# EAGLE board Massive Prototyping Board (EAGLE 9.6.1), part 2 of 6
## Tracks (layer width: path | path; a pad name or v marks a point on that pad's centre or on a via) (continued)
N$298  (via drill 0.94) (continued)
  Bottom 2.032: v80.01,48.26 v82.55,48.26 v85.09,48.26 v87.63,48.26 v90.17,48.26
N$299  (via drill 0.94)
  Bottom 2.032: v80.01,50.8 v82.55,50.8 v85.09,50.8 v87.63,50.8 v90.17,50.8
N$300  (via drill 0.94)
  Bottom 2.032: v80.01,53.34 v82.55,53.34 v85.09,53.34 v87.63,53.34 v90.17,53.34
N$301  (via drill 0.94)
  Bottom 2.032: v80.01,55.88 v82.55,55.88 v85.09,55.88 v87.63,55.88 v90.17,55.88
N$302  (via drill 0.94)
  Bottom 2.032: v80.01,58.42 v82.55,58.42 v85.09,58.42 v87.63,58.42 v90.17,58.42
N$303  (via drill 0.94)
  Bottom 2.032: v80.01,60.96 v82.55,60.96 v85.09,60.96 v87.63,60.96 v90.17,60.96
N$304  (via drill 0.94)
  Bottom 2.032: v80.01,63.5 v82.55,63.5 v85.09,63.5 v87.63,63.5 v90.17,63.5
N$305  (via drill 0.94)
  Bottom 2.032: v80.01,66.04 v82.55,66.04 v85.09,66.04 v87.63,66.04 v90.17,66.04
N$306  (via drill 0.94)
  Bottom 2.032: v80.01,68.58 v82.55,68.58 v85.09,68.58 v87.63,68.58 v90.17,68.58
N$307  (via drill 0.94)
  Bottom 2.032: v80.01,71.12 v82.55,71.12 v85.09,71.12 v87.63,71.12 v90.17,71.12
N$308  (via drill 0.94)
  Bottom 2.032: v80.01,73.66 v82.55,73.66 v85.09,73.66 v87.63,73.66 v90.17,73.66
N$309  (via drill 0.94)
  Bottom 2.032: v80.01,76.2 v82.55,76.2 v85.09,76.2 v87.63,76.2 v90.17,76.2
N$310  (via drill 0.94)
  Bottom 2.032: v80.01,78.74 v82.55,78.74 v85.09,78.74 v87.63,78.74 v90.17,78.74
N$311  (via drill 0.94)
  Bottom 2.032: v80.01,81.28 v82.55,81.28 v85.09,81.28 v87.63,81.28 v90.17,81.28
N$312  (via drill 0.94)
  Bottom 2.032: v80.01,83.82 v82.55,83.82 v85.09,83.82 v87.63,83.82 v90.17,83.82
N$313  (via drill 0.94)
  Bottom 2.032: v80.01,86.36 v82.55,86.36 v85.09,86.36 v87.63,86.36 v90.17,86.36
N$314  (via drill 0.94)
  Bottom 2.032: v80.01,88.9 v82.55,88.9 v85.09,88.9 v87.63,88.9 v90.17,88.9
N$315  (via drill 0.94)
  Bottom 2.032: v80.01,91.44 v82.55,91.44 v85.09,91.44 v87.63,91.44 v90.17,91.44
N$316  (via drill 0.94)
  Bottom 2.032: v80.01,93.98 v82.55,93.98 v85.09,93.98 v87.63,93.98 v90.17,93.98
N$317  (via drill 0.94)
  Bottom 2.032: v80.01,96.52 v82.55,96.52 v85.09,96.52 v87.63,96.52 v90.17,96.52
N$318  (via drill 0.94)
  Bottom 2.032: v80.01,99.06 v82.55,99.06 v85.09,99.06 v87.63,99.06 v90.17,99.06
N$319  (via drill 0.94)
  Bottom 2.032: v80.01,101.6 v82.55,101.6 v85.09,101.6 v87.63,101.6 v90.17,101.6
N$320  (via drill 0.94)
  Bottom 2.032: v80.01,104.14 v82.55,104.14 v85.09,104.14 v87.63,104.14 v90.17,104.14
N$321  (via drill 0.94)
  Bottom 2.032: v80.01,106.68 v82.55,106.68 v85.09,106.68 v87.63,106.68 v90.17,106.68
N$322  (via drill 0.94)
  Bottom 2.032: v80.01,109.22 v82.55,109.22 v85.09,109.22 v87.63,109.22 v90.17,109.22
N$323  (via drill 0.94)
  Bottom 2.032: v80.01,111.76 v82.55,111.76 v85.09,111.76 v87.63,111.76 v90.17,111.76
N$324  (via drill 0.94)
  Bottom 2.032: v80.01,114.3 v82.55,114.3 v85.09,114.3 v87.63,114.3 v90.17,114.3
N$325  (via drill 0.94)
  Bottom 2.032: v80.01,116.84 v82.55,116.84 v85.09,116.84 v87.63,116.84 v90.17,116.84
N$326  (via drill 0.94)
  Bottom 2.032: v80.01,119.38 v82.55,119.38 v85.09,119.38 v87.63,119.38 v90.17,119.38
N$327  (via drill 0.94)
  Bottom 2.032: v80.01,121.92 v82.55,121.92 v85.09,121.92 v87.63,121.92 v90.17,121.92
N$328  (via drill 0.94)
  Bottom 2.032: v80.01,124.46 v82.55,124.46 v85.09,124.46 v87.63,124.46 v90.17,124.46
N$329  (via drill 0.94)
  Bottom 2.032: v80.01,127 v82.55,127 v85.09,127 v87.63,127 v90.17,127
N$330  (via drill 0.94)
  Bottom 2.032: v80.01,129.54 v82.55,129.54 v85.09,129.54 v87.63,129.54 v90.17,129.54
N$331  (via drill 0.94)
  Bottom 2.032: v80.01,132.08 v82.55,132.08 v85.09,132.08 v87.63,132.08 v90.17,132.08
N$332  (via drill 0.94)
  Bottom 2.032: v80.01,134.62 v82.55,134.62 v85.09,134.62 v87.63,134.62 v90.17,134.62
N$333  (via drill 0.94)
  Bottom 2.032: v80.01,137.16 v82.55,137.16 v85.09,137.16 v87.63,137.16 v90.17,137.16
N$334  (via drill 0.94)
  Bottom 2.032: v80.01,139.7 v82.55,139.7 v85.09,139.7 v87.63,139.7 v90.17,139.7
N$335  (via drill 0.94)
  Bottom 2.032: v80.01,142.24 v82.55,142.24 v85.09,142.24 v87.63,142.24 v90.17,142.24
N$336  (via drill 0.94)
  Bottom 2.032: v80.01,144.78 v82.55,144.78 v85.09,144.78 v87.63,144.78 v90.17,144.78
N$337  (via drill 0.94)
  Bottom 2.032: v80.01,147.32 v82.55,147.32 v85.09,147.32 v87.63,147.32 v90.17,147.32
N$338  (via drill 0.94)
  Bottom 2.032: v80.01,149.86 v82.55,149.86 v85.09,149.86 v87.63,149.86 v90.17,149.86
N$339  (via drill 0.94)
  Bottom 2.032: v80.01,152.4 v82.55,152.4 v85.09,152.4 v87.63,152.4 v90.17,152.4
N$340  (via drill 0.94)
  Bottom 2.032: v80.01,154.94 v82.55,154.94 v85.09,154.94 v87.63,154.94 v90.17,154.94
N$341  (via drill 0.94)
  Bottom 2.032: v80.01,157.48 v82.55,157.48 v85.09,157.48 v87.63,157.48 v90.17,157.48
N$342  (via drill 0.94)
  Bottom 2.032: v80.01,160.02 v82.55,160.02 v85.09,160.02 v87.63,160.02 v90.17,160.02
N$343  (via drill 0.94)
  Bottom 2.032: v80.01,162.56 v82.55,162.56 v85.09,162.56 v87.63,162.56 v90.17,162.56
N$344  (via drill 0.94)
  Bottom 2.032: v80.01,165.1 v82.55,165.1 v85.09,165.1 v87.63,165.1 v90.17,165.1
N$345  (via drill 0.94)
  Bottom 2.032: v80.01,167.64 v82.55,167.64 v85.09,167.64 v87.63,167.64 v90.17,167.64
N$346  (via drill 0.94)
  Bottom 2.032: v80.01,170.18 v82.55,170.18 v85.09,170.18 v87.63,170.18 v90.17,170.18
N$347  (via drill 0.94)
  Bottom 2.032: v80.01,172.72 v82.55,172.72 v85.09,172.72 v87.63,172.72 v90.17,172.72
N$348  (via drill 0.94)
  Bottom 2.032: v80.01,175.26 v82.55,175.26 v85.09,175.26 v87.63,175.26 v90.17,175.26
N$349  (via drill 0.94)
  Bottom 2.032: v80.01,177.8 v82.55,177.8 v85.09,177.8 v87.63,177.8 v90.17,177.8
N$350  (via drill 0.94)
  Bottom 2.032: v80.01,180.34 v82.55,180.34 v85.09,180.34 v87.63,180.34 v90.17,180.34
N$351  (via drill 0.94)
  Bottom 2.032: v80.01,182.88 v82.55,182.88 v85.09,182.88 v87.63,182.88 v90.17,182.88
N$352  (via drill 0.94)
  Bottom 2.032: v80.01,185.42 v82.55,185.42 v85.09,185.42 v87.63,185.42 v90.17,185.42
N$353  (via drill 0.94)
  Bottom 2.032: v80.01,187.96 v82.55,187.96 v85.09,187.96 v87.63,187.96 v90.17,187.96
N$354  (via drill 0.94)
  Bottom 2.032: v80.01,190.5 v82.55,190.5 v85.09,190.5 v87.63,190.5 v90.17,190.5
N$355  (via drill 0.94)
  Bottom 2.032: v80.01,193.04 v82.55,193.04 v85.09,193.04 v87.63,193.04 v90.17,193.04
N$356  (via drill 0.94)
  Bottom 2.032: v80.01,195.58 v82.55,195.58 v85.09,195.58 v87.63,195.58 v90.17,195.58
N$357  (via drill 0.94)
  Bottom 2.032: v80.01,198.12 v82.55,198.12 v85.09,198.12 v87.63,198.12 v90.17,198.12
N$358  (via drill 0.94)
  Bottom 2.032: v80.01,200.66 v82.55,200.66 v85.09,200.66 v87.63,200.66 v90.17,200.66
N$359  (via drill 0.94)
  Bottom 2.032: v80.01,203.2 v82.55,203.2 v85.09,203.2 v87.63,203.2 v90.17,203.2
N$360  (via drill 0.94)
  Bottom 2.032: v80.01,205.74 v82.55,205.74 v85.09,205.74 v87.63,205.74 v90.17,205.74
N$361  (via drill 0.94)
  Bottom 2.032: v80.01,208.28 v82.55,208.28 v85.09,208.28 v87.63,208.28 v90.17,208.28
N$362  (via drill 0.94)
  Bottom 2.032: v80.01,210.82 v82.55,210.82 v85.09,210.82 v87.63,210.82 v90.17,210.82
N$363  (via drill 0.94)
  Bottom 2.032: v80.01,213.36 v82.55,213.36 v85.09,213.36 v87.63,213.36 v90.17,213.36
N$364  (via drill 0.94)
  Bottom 2.032: v80.01,215.9 v82.55,215.9 v85.09,215.9 v87.63,215.9 v90.17,215.9
N$365  (via drill 0.94)
  Bottom 2.032: v80.01,218.44 v82.55,218.44 v85.09,218.44 v87.63,218.44 v90.17,218.44
N$366  (via drill 0.94)
  Bottom 2.032: v80.01,220.98 v82.55,220.98 v85.09,220.98 v87.63,220.98 v90.17,220.98
N$367  (via drill 0.94)
  Bottom 2.032: v80.01,223.52 v82.55,223.52 v85.09,223.52 v87.63,223.52 v90.17,223.52
N$368  (via drill 0.94)
  Bottom 2.032: v80.01,226.06 v82.55,226.06 v85.09,226.06 v87.63,226.06 v90.17,226.06
N$369  (via drill 0.94)
  Bottom 2.032: v80.01,228.6 v82.55,228.6 v85.09,228.6 v87.63,228.6 v90.17,228.6
N$370  (via drill 0.94)
  Bottom 2.032: v80.01,231.14 v82.55,231.14 v85.09,231.14 v87.63,231.14 v90.17,231.14
N$371  (via drill 0.94)
  Bottom 2.032: v80.01,233.68 v82.55,233.68 v85.09,233.68 v87.63,233.68 v90.17,233.68
N$372  (via drill 0.94)
  Bottom 2.032: v80.01,236.22 v82.55,236.22 v85.09,236.22 v87.63,236.22 v90.17,236.22
N$373  (via drill 0.94)
  Bottom 2.032: v80.01,238.76 v82.55,238.76 v85.09,238.76 v87.63,238.76 v90.17,238.76
N$374  (via drill 0.94)
  Bottom 2.032: v80.01,241.3 v82.55,241.3 v85.09,241.3 v87.63,241.3 v90.17,241.3
N$375  (via drill 0.94)
  Bottom 2.032: v80.01,243.84 v82.55,243.84 v85.09,243.84 v87.63,243.84 v90.17,243.84
N$376  (via drill 0.94)
  Bottom 2.032: v80.01,246.38 v82.55,246.38 v85.09,246.38 v87.63,246.38 v90.17,246.38
N$377  (via drill 0.94)
  Bottom 2.032: v80.01,248.92 v82.55,248.92 v85.09,248.92 v87.63,248.92 v90.17,248.92
N$378  (via drill 0.94)
  Bottom 2.032: v80.01,251.46 v82.55,251.46 v85.09,251.46 v87.63,251.46 v90.17,251.46
N$379  (via drill 0.94)
  Bottom 2.032: v80.01,254 v82.55,254 v85.09,254 v87.63,254 v90.17,254
N$380  (via drill 0.94)
  Bottom 2.032: v80.01,256.54 v82.55,256.54 v85.09,256.54 v87.63,256.54 v90.17,256.54
N$381  (via drill 0.94)
  Bottom 2.032: v80.01,259.08 v82.55,259.08 v85.09,259.08 v87.63,259.08 v90.17,259.08
N$382  (via drill 0.94)
  Bottom 2.032: v80.01,261.62 v82.55,261.62 v85.09,261.62 v87.63,261.62 v90.17,261.62
N$383  (via drill 0.94)
  Bottom 2.032: v80.01,264.16 v82.55,264.16 v85.09,264.16 v87.63,264.16 v90.17,264.16
N$384  (via drill 0.94)
  Bottom 2.032: v80.01,266.7 v82.55,266.7 v85.09,266.7 v87.63,266.7 v90.17,266.7
N$385  (via drill 0.94)
  Bottom 2.032: v80.01,269.24 v82.55,269.24 v85.09,269.24 v87.63,269.24 v90.17,269.24
N$386  (via drill 0.94)
  Bottom 2.032: v80.01,271.78 v82.55,271.78 v85.09,271.78 v87.63,271.78 v90.17,271.78
N$387  (via drill 0.94)
  Bottom 2.032: v80.01,274.32 v82.55,274.32 v85.09,274.32 v87.63,274.32 v90.17,274.32
N$388  (via drill 0.94)
  Bottom 2.032: v80.01,276.86 v82.55,276.86 v85.09,276.86 v87.63,276.86 v90.17,276.86
N$389  (via drill 0.94)
  Bottom 2.032: v97.79,12.7 v100.33,12.7 v102.87,12.7 v105.41,12.7 v107.95,12.7
N$390  (via drill 0.94)
  Bottom 2.032: v97.79,15.24 v100.33,15.24 v102.87,15.24 v105.41,15.24 v107.95,15.24
N$391  (via drill 0.94)
  Bottom 2.032: v97.79,17.78 v100.33,17.78 v102.87,17.78 v105.41,17.78 v107.95,17.78
N$392  (via drill 0.94)
  Bottom 2.032: v97.79,20.32 v100.33,20.32 v102.87,20.32 v105.41,20.32 v107.95,20.32
N$393  (via drill 0.94)
  Bottom 2.032: v97.79,22.86 v100.33,22.86 v102.87,22.86 v105.41,22.86 v107.95,22.86
N$394  (via drill 0.94)
  Bottom 2.032: v97.79,25.4 v100.33,25.4 v102.87,25.4 v105.41,25.4 v107.95,25.4
N$395  (via drill 0.94)
  Bottom 2.032: v97.79,27.94 v100.33,27.94 v102.87,27.94 v105.41,27.94 v107.95,27.94
N$396  (via drill 0.94)
  Bottom 2.032: v97.79,30.48 v100.33,30.48 v102.87,30.48 v105.41,30.48 v107.95,30.48
N$397  (via drill 0.94)
  Bottom 2.032: v97.79,33.02 v100.33,33.02 v102.87,33.02 v105.41,33.02 v107.95,33.02
N$398  (via drill 0.94)
  Bottom 2.032: v97.79,35.56 v100.33,35.56 v102.87,35.56 v105.41,35.56 v107.95,35.56
N$399  (via drill 0.94)
  Bottom 2.032: v97.79,38.1 v100.33,38.1 v102.87,38.1 v105.41,38.1 v107.95,38.1
N$400  (via drill 0.94)
  Bottom 2.032: v97.79,40.64 v100.33,40.64 v102.87,40.64 v105.41,40.64 v107.95,40.64
N$401  (via drill 0.94)
  Bottom 2.032: v97.79,43.18 v100.33,43.18 v102.87,43.18 v105.41,43.18 v107.95,43.18
N$402  (via drill 0.94)
  Bottom 2.032: v97.79,45.72 v100.33,45.72 v102.87,45.72 v105.41,45.72 v107.95,45.72
N$403  (via drill 0.94)
  Bottom 2.032: v97.79,48.26 v100.33,48.26 v102.87,48.26 v105.41,48.26 v107.95,48.26
N$404  (via drill 0.94)
  Bottom 2.032: v97.79,50.8 v100.33,50.8 v102.87,50.8 v105.41,50.8 v107.95,50.8
N$405  (via drill 0.94)
  Bottom 2.032: v97.79,53.34 v100.33,53.34 v102.87,53.34 v105.41,53.34 v107.95,53.34
N$406  (via drill 0.94)
  Bottom 2.032: v97.79,55.88 v100.33,55.88 v102.87,55.88 v105.41,55.88 v107.95,55.88
N$407  (via drill 0.94)
  Bottom 2.032: v97.79,58.42 v100.33,58.42 v102.87,58.42 v105.41,58.42 v107.95,58.42
N$408  (via drill 0.94)
  Bottom 2.032: v97.79,60.96 v100.33,60.96 v102.87,60.96 v105.41,60.96 v107.95,60.96
N$409  (via drill 0.94)
  Bottom 2.032: v97.79,63.5 v100.33,63.5 v102.87,63.5 v105.41,63.5 v107.95,63.5
N$410  (via drill 0.94)
  Bottom 2.032: v97.79,66.04 v100.33,66.04 v102.87,66.04 v105.41,66.04 v107.95,66.04
N$411  (via drill 0.94)
  Bottom 2.032: v97.79,68.58 v100.33,68.58 v102.87,68.58 v105.41,68.58 v107.95,68.58
N$412  (via drill 0.94)
  Bottom 2.032: v97.79,71.12 v100.33,71.12 v102.87,71.12 v105.41,71.12 v107.95,71.12
N$413  (via drill 0.94)
  Bottom 2.032: v97.79,73.66 v100.33,73.66 v102.87,73.66 v105.41,73.66 v107.95,73.66
N$414  (via drill 0.94)
  Bottom 2.032: v97.79,76.2 v100.33,76.2 v102.87,76.2 v105.41,76.2 v107.95,76.2
N$415  (via drill 0.94)
  Bottom 2.032: v97.79,78.74 v100.33,78.74 v102.87,78.74 v105.41,78.74 v107.95,78.74
N$416  (via drill 0.94)
  Bottom 2.032: v97.79,81.28 v100.33,81.28 v102.87,81.28 v105.41,81.28 v107.95,81.28
N$417  (via drill 0.94)
  Bottom 2.032: v97.79,83.82 v100.33,83.82 v102.87,83.82 v105.41,83.82 v107.95,83.82
N$418  (via drill 0.94)
  Bottom 2.032: v97.79,86.36 v100.33,86.36 v102.87,86.36 v105.41,86.36 v107.95,86.36
N$419  (via drill 0.94)
  Bottom 2.032: v97.79,88.9 v100.33,88.9 v102.87,88.9 v105.41,88.9 v107.95,88.9
N$420  (via drill 0.94)
  Bottom 2.032: v97.79,91.44 v100.33,91.44 v102.87,91.44 v105.41,91.44 v107.95,91.44
N$421  (via drill 0.94)
  Bottom 2.032: v97.79,93.98 v100.33,93.98 v102.87,93.98 v105.41,93.98 v107.95,93.98
N$422  (via drill 0.94)
  Bottom 2.032: v97.79,96.52 v100.33,96.52 v102.87,96.52 v105.41,96.52 v107.95,96.52
N$423  (via drill 0.94)
  Bottom 2.032: v97.79,99.06 v100.33,99.06 v102.87,99.06 v105.41,99.06 v107.95,99.06
N$424  (via drill 0.94)
  Bottom 2.032: v97.79,101.6 v100.33,101.6 v102.87,101.6 v105.41,101.6 v107.95,101.6
N$425  (via drill 0.94)
  Bottom 2.032: v97.79,104.14 v100.33,104.14 v102.87,104.14 v105.41,104.14 v107.95,104.14
N$426  (via drill 0.94)
  Bottom 2.032: v97.79,106.68 v100.33,106.68 v102.87,106.68 v105.41,106.68 v107.95,106.68
N$427  (via drill 0.94)
  Bottom 2.032: v97.79,109.22 v100.33,109.22 v102.87,109.22 v105.41,109.22 v107.95,109.22
N$428  (via drill 0.94)
  Bottom 2.032: v97.79,111.76 v100.33,111.76 v102.87,111.76 v105.41,111.76 v107.95,111.76
N$429  (via drill 0.94)
  Bottom 2.032: v97.79,114.3 v100.33,114.3 v102.87,114.3 v105.41,114.3 v107.95,114.3
N$430  (via drill 0.94)
  Bottom 2.032: v97.79,116.84 v100.33,116.84 v102.87,116.84 v105.41,116.84 v107.95,116.84
N$431  (via drill 0.94)
  Bottom 2.032: v97.79,119.38 v100.33,119.38 v102.87,119.38 v105.41,119.38 v107.95,119.38
N$432  (via drill 0.94)
  Bottom 2.032: v97.79,121.92 v100.33,121.92 v102.87,121.92 v105.41,121.92 v107.95,121.92
N$433  (via drill 0.94)
  Bottom 2.032: v97.79,124.46 v100.33,124.46 v102.87,124.46 v105.41,124.46 v107.95,124.46
N$434  (via drill 0.94)
  Bottom 2.032: v97.79,127 v100.33,127 v102.87,127 v105.41,127 v107.95,127
N$435  (via drill 0.94)
  Bottom 2.032: v97.79,129.54 v100.33,129.54 v102.87,129.54 v105.41,129.54 v107.95,129.54
N$436  (via drill 0.94)
  Bottom 2.032: v97.79,132.08 v100.33,132.08 v102.87,132.08 v105.41,132.08 v107.95,132.08
N$437  (via drill 0.94)
  Bottom 2.032: v97.79,134.62 v100.33,134.62 v102.87,134.62 v105.41,134.62 v107.95,134.62
N$438  (via drill 0.94)
  Bottom 2.032: v97.79,137.16 v100.33,137.16 v102.87,137.16 v105.41,137.16 v107.95,137.16
N$439  (via drill 0.94)
  Bottom 2.032: v97.79,139.7 v100.33,139.7 v102.87,139.7 v105.41,139.7 v107.95,139.7
N$440  (via drill 0.94)
  Bottom 2.032: v97.79,142.24 v100.33,142.24 v102.87,142.24 v105.41,142.24 v107.95,142.24
N$441  (via drill 0.94)
  Bottom 2.032: v97.79,144.78 v100.33,144.78 v102.87,144.78 v105.41,144.78 v107.95,144.78
N$442  (via drill 0.94)
  Bottom 2.032: v97.79,147.32 v100.33,147.32 v102.87,147.32 v105.41,147.32 v107.95,147.32
N$443  (via drill 0.94)
  Bottom 2.032: v97.79,149.86 v100.33,149.86 v102.87,149.86 v105.41,149.86 v107.95,149.86
N$444  (via drill 0.94)
  Bottom 2.032: v97.79,152.4 v100.33,152.4 v102.87,152.4 v105.41,152.4 v107.95,152.4
N$445  (via drill 0.94)
  Bottom 2.032: v97.79,154.94 v100.33,154.94 v102.87,154.94 v105.41,154.94 v107.95,154.94
N$446  (via drill 0.94)
  Bottom 2.032: v97.79,157.48 v100.33,157.48 v102.87,157.48 v105.41,157.48 v107.95,157.48
N$447  (via drill 0.94)
  Bottom 2.032: v97.79,160.02 v100.33,160.02 v102.87,160.02 v105.41,160.02 v107.95,160.02
N$448  (via drill 0.94)
  Bottom 2.032: v97.79,162.56 v100.33,162.56 v102.87,162.56 v105.41,162.56 v107.95,162.56
N$449  (via drill 0.94)
  Bottom 2.032: v97.79,165.1 v100.33,165.1 v102.87,165.1 v105.41,165.1 v107.95,165.1
N$450  (via drill 0.94)
  Bottom 2.032: v97.79,167.64 v100.33,167.64 v102.87,167.64 v105.41,167.64 v107.95,167.64
N$451  (via drill 0.94)
  Bottom 2.032: v97.79,170.18 v100.33,170.18 v102.87,170.18 v105.41,170.18 v107.95,170.18
N$452  (via drill 0.94)
  Bottom 2.032: v97.79,172.72 v100.33,172.72 v102.87,172.72 v105.41,172.72 v107.95,172.72
N$453  (via drill 0.94)
  Bottom 2.032: v97.79,175.26 v100.33,175.26 v102.87,175.26 v105.41,175.26 v107.95,175.26
N$454  (via drill 0.94)
  Bottom 2.032: v97.79,177.8 v100.33,177.8 v102.87,177.8 v105.41,177.8 v107.95,177.8
N$455  (via drill 0.94)
  Bottom 2.032: v97.79,180.34 v100.33,180.34 v102.87,180.34 v105.41,180.34 v107.95,180.34
N$456  (via drill 0.94)
  Bottom 2.032: v97.79,182.88 v100.33,182.88 v102.87,182.88 v105.41,182.88 v107.95,182.88
N$457  (via drill 0.94)
  Bottom 2.032: v97.79,185.42 v100.33,185.42 v102.87,185.42 v105.41,185.42 v107.95,185.42
N$458  (via drill 0.94)
  Bottom 2.032: v97.79,187.96 v100.33,187.96 v102.87,187.96 v105.41,187.96 v107.95,187.96
N$459  (via drill 0.94)
  Bottom 2.032: v97.79,190.5 v100.33,190.5 v102.87,190.5 v105.41,190.5 v107.95,190.5
N$460  (via drill 0.94)
  Bottom 2.032: v97.79,193.04 v100.33,193.04 v102.87,193.04 v105.41,193.04 v107.95,193.04
N$461  (via drill 0.94)
  Bottom 2.032: v97.79,195.58 v100.33,195.58 v102.87,195.58 v105.41,195.58 v107.95,195.58
N$462  (via drill 0.94)
  Bottom 2.032: v97.79,198.12 v100.33,198.12 v102.87,198.12 v105.41,198.12 v107.95,198.12
N$463  (via drill 0.94)
  Bottom 2.032: v97.79,200.66 v100.33,200.66 v102.87,200.66 v105.41,200.66 v107.95,200.66
N$464  (via drill 0.94)
  Bottom 2.032: v97.79,203.2 v100.33,203.2 v102.87,203.2 v105.41,203.2 v107.95,203.2
N$465  (via drill 0.94)
  Bottom 2.032: v97.79,205.74 v100.33,205.74 v102.87,205.74 v105.41,205.74 v107.95,205.74
N$466  (via drill 0.94)
  Bottom 2.032: v97.79,208.28 v100.33,208.28 v102.87,208.28 v105.41,208.28 v107.95,208.28
N$467  (via drill 0.94)
  Bottom 2.032: v97.79,210.82 v100.33,210.82 v102.87,210.82 v105.41,210.82 v107.95,210.82
N$468  (via drill 0.94)
  Bottom 2.032: v97.79,213.36 v100.33,213.36 v102.87,213.36 v105.41,213.36 v107.95,213.36
N$469  (via drill 0.94)
  Bottom 2.032: v97.79,215.9 v100.33,215.9 v102.87,215.9 v105.41,215.9 v107.95,215.9
N$470  (via drill 0.94)
  Bottom 2.032: v97.79,218.44 v100.33,218.44 v102.87,218.44 v105.41,218.44 v107.95,218.44
N$471  (via drill 0.94)
  Bottom 2.032: v97.79,220.98 v100.33,220.98 v102.87,220.98 v105.41,220.98 v107.95,220.98
N$472  (via drill 0.94)
  Bottom 2.032: v97.79,223.52 v100.33,223.52 v102.87,223.52 v105.41,223.52 v107.95,223.52
N$473  (via drill 0.94)
  Bottom 2.032: v97.79,226.06 v100.33,226.06 v102.87,226.06 v105.41,226.06 v107.95,226.06
N$474  (via drill 0.94)
  Bottom 2.032: v97.79,228.6 v100.33,228.6 v102.87,228.6 v105.41,228.6 v107.95,228.6
N$475  (via drill 0.94)
  Bottom 2.032: v97.79,231.14 v100.33,231.14 v102.87,231.14 v105.41,231.14 v107.95,231.14
N$476  (via drill 0.94)
  Bottom 2.032: v97.79,233.68 v100.33,233.68 v102.87,233.68 v105.41,233.68 v107.95,233.68
N$477  (via drill 0.94)
  Bottom 2.032: v97.79,236.22 v100.33,236.22 v102.87,236.22 v105.41,236.22 v107.95,236.22
N$478  (via drill 0.94)
  Bottom 2.032: v97.79,238.76 v100.33,238.76 v102.87,238.76 v105.41,238.76 v107.95,238.76
N$479  (via drill 0.94)
  Bottom 2.032: v97.79,241.3 v100.33,241.3 v102.87,241.3 v105.41,241.3 v107.95,241.3
N$480  (via drill 0.94)
  Bottom 2.032: v97.79,243.84 v100.33,243.84 v102.87,243.84 v105.41,243.84 v107.95,243.84
N$481  (via drill 0.94)
  Bottom 2.032: v97.79,246.38 v100.33,246.38 v102.87,246.38 v105.41,246.38 v107.95,246.38
N$482  (via drill 0.94)
  Bottom 2.032: v97.79,248.92 v100.33,248.92 v102.87,248.92 v105.41,248.92 v107.95,248.92
N$483  (via drill 0.94)
  Bottom 2.032: v97.79,251.46 v100.33,251.46 v102.87,251.46 v105.41,251.46 v107.95,251.46
N$484  (via drill 0.94)
  Bottom 2.032: v97.79,254 v100.33,254 v102.87,254 v105.41,254 v107.95,254
N$485  (via drill 0.94)
  Bottom 2.032: v97.79,256.54 v100.33,256.54 v102.87,256.54 v105.41,256.54 v107.95,256.54
N$486  (via drill 0.94)
  Bottom 2.032: v97.79,259.08 v100.33,259.08 v102.87,259.08 v105.41,259.08 v107.95,259.08
N$487  (via drill 0.94)
  Bottom 2.032: v97.79,261.62 v100.33,261.62 v102.87,261.62 v105.41,261.62 v107.95,261.62
N$488  (via drill 0.94)
  Bottom 2.032: v97.79,264.16 v100.33,264.16 v102.87,264.16 v105.41,264.16 v107.95,264.16
N$489  (via drill 0.94)
  Bottom 2.032: v97.79,266.7 v100.33,266.7 v102.87,266.7 v105.41,266.7 v107.95,266.7
N$490  (via drill 0.94)
  Bottom 2.032: v97.79,269.24 v100.33,269.24 v102.87,269.24 v105.41,269.24 v107.95,269.24
N$491  (via drill 0.94)
  Bottom 2.032: v97.79,271.78 v100.33,271.78 v102.87,271.78 v105.41,271.78 v107.95,271.78
N$492  (via drill 0.94)
  Bottom 2.032: v97.79,274.32 v100.33,274.32 v102.87,274.32 v105.41,274.32 v107.95,274.32
N$493  (via drill 0.94)
  Bottom 2.032: v97.79,276.86 v100.33,276.86 v102.87,276.86 v105.41,276.86 v107.95,276.86
N$494  (via drill 0.94)
  Bottom 2.032: v110.49,12.7 v113.03,12.7 v115.57,12.7 v118.11,12.7 v120.65,12.7
N$495  (via drill 0.94)
  Bottom 2.032: v110.49,15.24 v113.03,15.24 v115.57,15.24 v118.11,15.24 v120.65,15.24
N$496  (via drill 0.94)
  Bottom 2.032: v110.49,17.78 v113.03,17.78 v115.57,17.78 v118.11,17.78 v120.65,17.78
N$497  (via drill 0.94)
  Bottom 2.032: v110.49,20.32 v113.03,20.32 v115.57,20.32 v118.11,20.32 v120.65,20.32
N$498  (via drill 0.94)
  Bottom 2.032: v110.49,22.86 v113.03,22.86 v115.57,22.86 v118.11,22.86 v120.65,22.86
N$499  (via drill 0.94)
  Bottom 2.032: v110.49,25.4 v113.03,25.4 v115.57,25.4 v118.11,25.4 v120.65,25.4
N$500  (via drill 0.94)
  Bottom 2.032: v110.49,27.94 v113.03,27.94 v115.57,27.94 v118.11,27.94 v120.65,27.94
N$501  (via drill 0.94)
  Bottom 2.032: v110.49,30.48 v113.03,30.48 v115.57,30.48 v118.11,30.48 v120.65,30.48
N$502  (via drill 0.94)
  Bottom 2.032: v110.49,33.02 v113.03,33.02 v115.57,33.02 v118.11,33.02 v120.65,33.02
N$503  (via drill 0.94)
  Bottom 2.032: v110.49,35.56 v113.03,35.56 v115.57,35.56 v118.11,35.56 v120.65,35.56
N$504  (via drill 0.94)
  Bottom 2.032: v110.49,38.1 v113.03,38.1 v115.57,38.1 v118.11,38.1 v120.65,38.1
N$505  (via drill 0.94)
  Bottom 2.032: v110.49,40.64 v113.03,40.64 v115.57,40.64 v118.11,40.64 v120.65,40.64
N$506  (via drill 0.94)
  Bottom 2.032: v110.49,43.18 v113.03,43.18 v115.57,43.18 v118.11,43.18 v120.65,43.18
N$507  (via drill 0.94)
  Bottom 2.032: v110.49,45.72 v113.03,45.72 v115.57,45.72 v118.11,45.72 v120.65,45.72
N$508  (via drill 0.94)
  Bottom 2.032: v110.49,48.26 v113.03,48.26 v115.57,48.26 v118.11,48.26 v120.65,48.26
N$509  (via drill 0.94)
  Bottom 2.032: v110.49,50.8 v113.03,50.8 v115.57,50.8 v118.11,50.8 v120.65,50.8
N$510  (via drill 0.94)
  Bottom 2.032: v110.49,53.34 v113.03,53.34 v115.57,53.34 v118.11,53.34 v120.65,53.34
N$511  (via drill 0.94)
  Bottom 2.032: v110.49,55.88 v113.03,55.88 v115.57,55.88 v118.11,55.88 v120.65,55.88
N$512  (via drill 0.94)
  Bottom 2.032: v110.49,58.42 v113.03,58.42 v115.57,58.42 v118.11,58.42 v120.65,58.42
N$513  (via drill 0.94)
  Bottom 2.032: v110.49,60.96 v113.03,60.96 v115.57,60.96 v118.11,60.96 v120.65,60.96
N$514  (via drill 0.94)
  Bottom 2.032: v110.49,63.5 v113.03,63.5 v115.57,63.5 v118.11,63.5 v120.65,63.5
N$515  (via drill 0.94)
  Bottom 2.032: v110.49,66.04 v113.03,66.04 v115.57,66.04 v118.11,66.04 v120.65,66.04
N$516  (via drill 0.94)
  Bottom 2.032: v110.49,68.58 v113.03,68.58 v115.57,68.58 v118.11,68.58 v120.65,68.58
N$517  (via drill 0.94)
  Bottom 2.032: v110.49,71.12 v113.03,71.12 v115.57,71.12 v118.11,71.12 v120.65,71.12
N$518  (via drill 0.94)
  Bottom 2.032: v110.49,73.66 v113.03,73.66 v115.57,73.66 v118.11,73.66 v120.65,73.66
N$519  (via drill 0.94)
  Bottom 2.032: v110.49,76.2 v113.03,76.2 v115.57,76.2 v118.11,76.2 v120.65,76.2
N$520  (via drill 0.94)
  Bottom 2.032: v110.49,78.74 v113.03,78.74 v115.57,78.74 v118.11,78.74 v120.65,78.74
N$521  (via drill 0.94)
  Bottom 2.032: v110.49,81.28 v113.03,81.28 v115.57,81.28 v118.11,81.28 v120.65,81.28
N$522  (via drill 0.94)
  Bottom 2.032: v110.49,83.82 v113.03,83.82 v115.57,83.82 v118.11,83.82 v120.65,83.82
N$523  (via drill 0.94)
  Bottom 2.032: v110.49,86.36 v113.03,86.36 v115.57,86.36 v118.11,86.36 v120.65,86.36
N$524  (via drill 0.94)
  Bottom 2.032: v110.49,88.9 v113.03,88.9 v115.57,88.9 v118.11,88.9 v120.65,88.9
N$525  (via drill 0.94)
  Bottom 2.032: v110.49,91.44 v113.03,91.44 v115.57,91.44 v118.11,91.44 v120.65,91.44
N$526  (via drill 0.94)
  Bottom 2.032: v110.49,93.98 v113.03,93.98 v115.57,93.98 v118.11,93.98 v120.65,93.98
N$527  (via drill 0.94)
  Bottom 2.032: v110.49,96.52 v113.03,96.52 v115.57,96.52 v118.11,96.52 v120.65,96.52
N$528  (via drill 0.94)
  Bottom 2.032: v110.49,99.06 v113.03,99.06 v115.57,99.06 v118.11,99.06 v120.65,99.06
N$529  (via drill 0.94)
  Bottom 2.032: v110.49,101.6 v113.03,101.6 v115.57,101.6 v118.11,101.6 v120.65,101.6
N$530  (via drill 0.94)
  Bottom 2.032: v110.49,104.14 v113.03,104.14 v115.57,104.14 v118.11,104.14 v120.65,104.14
N$531  (via drill 0.94)
  Bottom 2.032: v110.49,106.68 v113.03,106.68 v115.57,106.68 v118.11,106.68 v120.65,106.68
N$532  (via drill 0.94)
  Bottom 2.032: v110.49,109.22 v113.03,109.22 v115.57,109.22 v118.11,109.22 v120.65,109.22
N$533  (via drill 0.94)
  Bottom 2.032: v110.49,111.76 v113.03,111.76 v115.57,111.76 v118.11,111.76 v120.65,111.76
N$534  (via drill 0.94)
  Bottom 2.032: v110.49,114.3 v113.03,114.3 v115.57,114.3 v118.11,114.3 v120.65,114.3
N$535  (via drill 0.94)
  Bottom 2.032: v110.49,116.84 v113.03,116.84 v115.57,116.84 v118.11,116.84 v120.65,116.84
N$536  (via drill 0.94)
  Bottom 2.032: v110.49,119.38 v113.03,119.38 v115.57,119.38 v118.11,119.38 v120.65,119.38
N$537  (via drill 0.94)
  Bottom 2.032: v110.49,121.92 v113.03,121.92 v115.57,121.92 v118.11,121.92 v120.65,121.92
N$538  (via drill 0.94)
  Bottom 2.032: v110.49,124.46 v113.03,124.46 v115.57,124.46 v118.11,124.46 v120.65,124.46
N$539  (via drill 0.94)
  Bottom 2.032: v110.49,127 v113.03,127 v115.57,127 v118.11,127 v120.65,127
N$540  (via drill 0.94)
  Bottom 2.032: v110.49,129.54 v113.03,129.54 v115.57,129.54 v118.11,129.54 v120.65,129.54
N$541  (via drill 0.94)
  Bottom 2.032: v110.49,132.08 v113.03,132.08 v115.57,132.08 v118.11,132.08 v120.65,132.08
N$542  (via drill 0.94)
  Bottom 2.032: v110.49,134.62 v113.03,134.62 v115.57,134.62 v118.11,134.62 v120.65,134.62
N$543  (via drill 0.94)
  Bottom 2.032: v110.49,137.16 v113.03,137.16 v115.57,137.16 v118.11,137.16 v120.65,137.16
N$544  (via drill 0.94)
  Bottom 2.032: v110.49,139.7 v113.03,139.7 v115.57,139.7 v118.11,139.7 v120.65,139.7
N$545  (via drill 0.94)
  Bottom 2.032: v110.49,142.24 v113.03,142.24 v115.57,142.24 v118.11,142.24 v120.65,142.24
N$546  (via drill 0.94)
  Bottom 2.032: v110.49,144.78 v113.03,144.78 v115.57,144.78 v118.11,144.78 v120.65,144.78
N$547  (via drill 0.94)
  Bottom 2.032: v110.49,147.32 v113.03,147.32 v115.57,147.32 v118.11,147.32 v120.65,147.32
N$548  (via drill 0.94)
  Bottom 2.032: v110.49,149.86 v113.03,149.86 v115.57,149.86 v118.11,149.86 v120.65,149.86
N$549  (via drill 0.94)
  Bottom 2.032: v110.49,152.4 v113.03,152.4 v115.57,152.4 v118.11,152.4 v120.65,152.4
N$550  (via drill 0.94)
  Bottom 2.032: v110.49,154.94 v113.03,154.94 v115.57,154.94 v118.11,154.94 v120.65,154.94
N$551  (via drill 0.94)
  Bottom 2.032: v110.49,157.48 v113.03,157.48 v115.57,157.48 v118.11,157.48 v120.65,157.48
N$552  (via drill 0.94)
  Bottom 2.032: v110.49,160.02 v113.03,160.02 v115.57,160.02 v118.11,160.02 v120.65,160.02
N$553  (via drill 0.94)
  Bottom 2.032: v110.49,162.56 v113.03,162.56 v115.57,162.56 v118.11,162.56 v120.65,162.56
N$554  (via drill 0.94)
  Bottom 2.032: v110.49,165.1 v113.03,165.1 v115.57,165.1 v118.11,165.1 v120.65,165.1
N$555  (via drill 0.94)
  Bottom 2.032: v110.49,167.64 v113.03,167.64 v115.57,167.64 v118.11,167.64 v120.65,167.64
N$556  (via drill 0.94)
  Bottom 2.032: v110.49,170.18 v113.03,170.18 v115.57,170.18 v118.11,170.18 v120.65,170.18
N$557  (via drill 0.94)
  Bottom 2.032: v110.49,172.72 v113.03,172.72 v115.57,172.72 v118.11,172.72 v120.65,172.72
N$558  (via drill 0.94)
  Bottom 2.032: v110.49,175.26 v113.03,175.26 v115.57,175.26 v118.11,175.26 v120.65,175.26
N$559  (via drill 0.94)
  Bottom 2.032: v110.49,177.8 v113.03,177.8 v115.57,177.8 v118.11,177.8 v120.65,177.8
N$560  (via drill 0.94)
  Bottom 2.032: v110.49,180.34 v113.03,180.34 v115.57,180.34 v118.11,180.34 v120.65,180.34
N$561  (via drill 0.94)
  Bottom 2.032: v110.49,182.88 v113.03,182.88 v115.57,182.88 v118.11,182.88 v120.65,182.88
N$562  (via drill 0.94)
  Bottom 2.032: v110.49,185.42 v113.03,185.42 v115.57,185.42 v118.11,185.42 v120.65,185.42
N$563  (via drill 0.94)
  Bottom 2.032: v110.49,187.96 v113.03,187.96 v115.57,187.96 v118.11,187.96 v120.65,187.96
N$564  (via drill 0.94)
  Bottom 2.032: v110.49,190.5 v113.03,190.5 v115.57,190.5 v118.11,190.5 v120.65,190.5
N$565  (via drill 0.94)
  Bottom 2.032: v110.49,193.04 v113.03,193.04 v115.57,193.04 v118.11,193.04 v120.65,193.04
N$566  (via drill 0.94)
  Bottom 2.032: v110.49,195.58 v113.03,195.58 v115.57,195.58 v118.11,195.58 v120.65,195.58
N$567  (via drill 0.94)
  Bottom 2.032: v110.49,198.12 v113.03,198.12 v115.57,198.12 v118.11,198.12 v120.65,198.12
N$568  (via drill 0.94)
  Bottom 2.032: v110.49,200.66 v113.03,200.66 v115.57,200.66 v118.11,200.66 v120.65,200.66
N$569  (via drill 0.94)
  Bottom 2.032: v110.49,203.2 v113.03,203.2 v115.57,203.2 v118.11,203.2 v120.65,203.2
N$570  (via drill 0.94)
  Bottom 2.032: v110.49,205.74 v113.03,205.74 v115.57,205.74 v118.11,205.74 v120.65,205.74
N$571  (via drill 0.94)
  Bottom 2.032: v110.49,208.28 v113.03,208.28 v115.57,208.28 v118.11,208.28 v120.65,208.28
N$572  (via drill 0.94)
  Bottom 2.032: v110.49,210.82 v113.03,210.82 v115.57,210.82 v118.11,210.82 v120.65,210.82
N$573  (via drill 0.94)
  Bottom 2.032: v110.49,213.36 v113.03,213.36 v115.57,213.36 v118.11,213.36 v120.65,213.36
N$574  (via drill 0.94)
  Bottom 2.032: v110.49,215.9 v113.03,215.9 v115.57,215.9 v118.11,215.9 v120.65,215.9
N$575  (via drill 0.94)
  Bottom 2.032: v110.49,218.44 v113.03,218.44 v115.57,218.44 v118.11,218.44 v120.65,218.44
N$576  (via drill 0.94)
  Bottom 2.032: v110.49,220.98 v113.03,220.98 v115.57,220.98 v118.11,220.98 v120.65,220.98
N$577  (via drill 0.94)
  Bottom 2.032: v110.49,223.52 v113.03,223.52 v115.57,223.52 v118.11,223.52 v120.65,223.52
N$578  (via drill 0.94)
  Bottom 2.032: v110.49,226.06 v113.03,226.06 v115.57,226.06 v118.11,226.06 v120.65,226.06
N$579  (via drill 0.94)
  Bottom 2.032: v110.49,228.6 v113.03,228.6 v115.57,228.6 v118.11,228.6 v120.65,228.6
N$580  (via drill 0.94)
  Bottom 2.032: v110.49,231.14 v113.03,231.14 v115.57,231.14 v118.11,231.14 v120.65,231.14
N$581  (via drill 0.94)
  Bottom 2.032: v110.49,233.68 v113.03,233.68 v115.57,233.68 v118.11,233.68 v120.65,233.68
N$582  (via drill 0.94)
  Bottom 2.032: v110.49,236.22 v113.03,236.22 v115.57,236.22 v118.11,236.22 v120.65,236.22
N$583  (via drill 0.94)
  Bottom 2.032: v110.49,238.76 v113.03,238.76 v115.57,238.76 v118.11,238.76 v120.65,238.76
N$584  (via drill 0.94)
  Bottom 2.032: v110.49,241.3 v113.03,241.3 v115.57,241.3 v118.11,241.3 v120.65,241.3
N$585  (via drill 0.94)
  Bottom 2.032: v110.49,243.84 v113.03,243.84 v115.57,243.84 v118.11,243.84 v120.65,243.84
N$586  (via drill 0.94)
  Bottom 2.032: v110.49,246.38 v113.03,246.38 v115.57,246.38 v118.11,246.38 v120.65,246.38
N$587  (via drill 0.94)
  Bottom 2.032: v110.49,248.92 v113.03,248.92 v115.57,248.92 v118.11,248.92 v120.65,248.92
N$588  (via drill 0.94)
  Bottom 2.032: v110.49,251.46 v113.03,251.46 v115.57,251.46 v118.11,251.46 v120.65,251.46
N$589  (via drill 0.94)
  Bottom 2.032: v110.49,254 v113.03,254 v115.57,254 v118.11,254 v120.65,254
N$590  (via drill 0.94)
  Bottom 2.032: v110.49,256.54 v113.03,256.54 v115.57,256.54 v118.11,256.54 v120.65,256.54
N$591  (via drill 0.94)
  Bottom 2.032: v110.49,259.08 v113.03,259.08 v115.57,259.08 v118.11,259.08 v120.65,259.08
N$592  (via drill 0.94)
  Bottom 2.032: v110.49,261.62 v113.03,261.62 v115.57,261.62 v118.11,261.62 v120.65,261.62
N$593  (via drill 0.94)
  Bottom 2.032: v110.49,264.16 v113.03,264.16 v115.57,264.16 v118.11,264.16 v120.65,264.16
N$594  (via drill 0.94)
  Bottom 2.032: v110.49,266.7 v113.03,266.7 v115.57,266.7 v118.11,266.7 v120.65,266.7
N$595  (via drill 0.94)
  Bottom 2.032: v110.49,269.24 v113.03,269.24 v115.57,269.24 v118.11,269.24 v120.65,269.24
N$596  (via drill 0.94)
  Bottom 2.032: v110.49,271.78 v113.03,271.78 v115.57,271.78 v118.11,271.78 v120.65,271.78
N$597  (via drill 0.94)
  Bottom 2.032: v110.49,274.32 v113.03,274.32 v115.57,274.32 v118.11,274.32 v120.65,274.32
N$598  (via drill 0.94)
  Bottom 2.032: v110.49,276.86 v113.03,276.86 v115.57,276.86 v118.11,276.86 v120.65,276.86
N$599  (via drill 0.94)
  Bottom 2.032: v128.27,12.7 v130.81,12.7 v133.35,12.7 v135.89,12.7 v138.43,12.7
N$600  (via drill 0.94)
  Bottom 2.032: v128.27,15.24 v130.81,15.24 v133.35,15.24 v135.89,15.24 v138.43,15.24
N$601  (via drill 0.94)
  Bottom 2.032: v128.27,17.78 v130.81,17.78 v133.35,17.78 v135.89,17.78 v138.43,17.78
N$602  (via drill 0.94)
  Bottom 2.032: v128.27,20.32 v130.81,20.32 v133.35,20.32 v135.89,20.32 v138.43,20.32
N$603  (via drill 0.94)
  Bottom 2.032: v128.27,22.86 v130.81,22.86 v133.35,22.86 v135.89,22.86 v138.43,22.86
N$604  (via drill 0.94)
  Bottom 2.032: v128.27,25.4 v130.81,25.4 v133.35,25.4 v135.89,25.4 v138.43,25.4
N$605  (via drill 0.94)
  Bottom 2.032: v128.27,27.94 v130.81,27.94 v133.35,27.94 v135.89,27.94 v138.43,27.94
N$606  (via drill 0.94)
  Bottom 2.032: v128.27,30.48 v130.81,30.48 v133.35,30.48 v135.89,30.48 v138.43,30.48
N$607  (via drill 0.94)
  Bottom 2.032: v128.27,33.02 v130.81,33.02 v133.35,33.02 v135.89,33.02 v138.43,33.02
N$608  (via drill 0.94)
  Bottom 2.032: v128.27,35.56 v130.81,35.56 v133.35,35.56 v135.89,35.56 v138.43,35.56
N$609  (via drill 0.94)
  Bottom 2.032: v128.27,38.1 v130.81,38.1 v133.35,38.1 v135.89,38.1 v138.43,38.1
N$610  (via drill 0.94)
  Bottom 2.032: v128.27,40.64 v130.81,40.64 v133.35,40.64 v135.89,40.64 v138.43,40.64
N$611  (via drill 0.94)
  Bottom 2.032: v128.27,43.18 v130.81,43.18 v133.35,43.18 v135.89,43.18 v138.43,43.18
N$612  (via drill 0.94)
  Bottom 2.032: v128.27,45.72 v130.81,45.72 v133.35,45.72 v135.89,45.72 v138.43,45.72
N$613  (via drill 0.94)
  Bottom 2.032: v128.27,48.26 v130.81,48.26 v133.35,48.26 v135.89,48.26 v138.43,48.26
N$614  (via drill 0.94)
  Bottom 2.032: v128.27,50.8 v130.81,50.8 v133.35,50.8 v135.89,50.8 v138.43,50.8
N$615  (via drill 0.94)
  Bottom 2.032: v128.27,53.34 v130.81,53.34 v133.35,53.34 v135.89,53.34 v138.43,53.34
N$616  (via drill 0.94)
  Bottom 2.032: v128.27,55.88 v130.81,55.88 v133.35,55.88 v135.89,55.88 v138.43,55.88
N$617  (via drill 0.94)
  Bottom 2.032: v128.27,58.42 v130.81,58.42 v133.35,58.42 v135.89,58.42 v138.43,58.42
N$618  (via drill 0.94)
  Bottom 2.032: v128.27,60.96 v130.81,60.96 v133.35,60.96 v135.89,60.96 v138.43,60.96
N$619  (via drill 0.94)
  Bottom 2.032: v128.27,63.5 v130.81,63.5 v133.35,63.5 v135.89,63.5 v138.43,63.5
N$620  (via drill 0.94)
  Bottom 2.032: v128.27,66.04 v130.81,66.04 v133.35,66.04 v135.89,66.04 v138.43,66.04
N$621  (via drill 0.94)
  Bottom 2.032: v128.27,68.58 v130.81,68.58 v133.35,68.58 v135.89,68.58 v138.43,68.58
N$622  (via drill 0.94)
  Bottom 2.032: v128.27,71.12 v130.81,71.12 v133.35,71.12 v135.89,71.12 v138.43,71.12
N$623  (via drill 0.94)
  Bottom 2.032: v128.27,73.66 v130.81,73.66 v133.35,73.66 v135.89,73.66 v138.43,73.66
N$624  (via drill 0.94)
  Bottom 2.032: v128.27,76.2 v130.81,76.2 v133.35,76.2 v135.89,76.2 v138.43,76.2
N$625  (via drill 0.94)
  Bottom 2.032: v128.27,78.74 v130.81,78.74 v133.35,78.74 v135.89,78.74 v138.43,78.74
N$626  (via drill 0.94)
  Bottom 2.032: v128.27,81.28 v130.81,81.28 v133.35,81.28 v135.89,81.28 v138.43,81.28
N$627  (via drill 0.94)
  Bottom 2.032: v128.27,83.82 v130.81,83.82 v133.35,83.82 v135.89,83.82 v138.43,83.82
N$628  (via drill 0.94)
  Bottom 2.032: v128.27,86.36 v130.81,86.36 v133.35,86.36 v135.89,86.36 v138.43,86.36
N$629  (via drill 0.94)
  Bottom 2.032: v128.27,88.9 v130.81,88.9 v133.35,88.9 v135.89,88.9 v138.43,88.9
N$630  (via drill 0.94)
  Bottom 2.032: v128.27,91.44 v130.81,91.44 v133.35,91.44 v135.89,91.44 v138.43,91.44
N$631  (via drill 0.94)
  Bottom 2.032: v128.27,93.98 v130.81,93.98 v133.35,93.98 v135.89,93.98 v138.43,93.98
N$632  (via drill 0.94)
  Bottom 2.032: v128.27,96.52 v130.81,96.52 v133.35,96.52 v135.89,96.52 v138.43,96.52
N$633  (via drill 0.94)
  Bottom 2.032: v128.27,99.06 v130.81,99.06 v133.35,99.06 v135.89,99.06 v138.43,99.06
N$634  (via drill 0.94)
  Bottom 2.032: v128.27,101.6 v130.81,101.6 v133.35,101.6 v135.89,101.6 v138.43,101.6
N$635  (via drill 0.94)
  Bottom 2.032: v128.27,104.14 v130.81,104.14 v133.35,104.14 v135.89,104.14 v138.43,104.14
N$636  (via drill 0.94)
  Bottom 2.032: v128.27,106.68 v130.81,106.68 v133.35,106.68 v135.89,106.68 v138.43,106.68
N$637  (via drill 0.94)
  Bottom 2.032: v128.27,109.22 v130.81,109.22 v133.35,109.22 v135.89,109.22 v138.43,109.22
N$638  (via drill 0.94)
  Bottom 2.032: v128.27,111.76 v130.81,111.76 v133.35,111.76 v135.89,111.76 v138.43,111.76
N$639  (via drill 0.94)
  Bottom 2.032: v128.27,114.3 v130.81,114.3 v133.35,114.3 v135.89,114.3 v138.43,114.3
N$640  (via drill 0.94)
  Bottom 2.032: v128.27,116.84 v130.81,116.84 v133.35,116.84 v135.89,116.84 v138.43,116.84
N$641  (via drill 0.94)
  Bottom 2.032: v128.27,119.38 v130.81,119.38 v133.35,119.38 v135.89,119.38 v138.43,119.38
N$642  (via drill 0.94)
  Bottom 2.032: v128.27,121.92 v130.81,121.92 v133.35,121.92 v135.89,121.92 v138.43,121.92
N$643  (via drill 0.94)
  Bottom 2.032: v128.27,124.46 v130.81,124.46 v133.35,124.46 v135.89,124.46 v138.43,124.46
N$644  (via drill 0.94)
  Bottom 2.032: v128.27,127 v130.81,127 v133.35,127 v135.89,127 v138.43,127
N$645  (via drill 0.94)
  Bottom 2.032: v128.27,129.54 v130.81,129.54 v133.35,129.54 v135.89,129.54 v138.43,129.54
N$646  (via drill 0.94)
  Bottom 2.032: v128.27,132.08 v130.81,132.08 v133.35,132.08 v135.89,132.08 v138.43,132.08
N$647  (via drill 0.94)
  Bottom 2.032: v128.27,134.62 v130.81,134.62 v133.35,134.62 v135.89,134.62 v138.43,134.62
N$648  (via drill 0.94)
  Bottom 2.032: v128.27,137.16 v130.81,137.16 v133.35,137.16 v135.89,137.16 v138.43,137.16
N$649  (via drill 0.94)
  Bottom 2.032: v128.27,139.7 v130.81,139.7 v133.35,139.7 v135.89,139.7 v138.43,139.7
N$650  (via drill 0.94)
  Bottom 2.032: v128.27,142.24 v130.81,142.24 v133.35,142.24 v135.89,142.24 v138.43,142.24
N$651  (via drill 0.94)
  Bottom 2.032: v128.27,144.78 v130.81,144.78 v133.35,144.78 v135.89,144.78 v138.43,144.78
N$652  (via drill 0.94)
  Bottom 2.032: v128.27,147.32 v130.81,147.32 v133.35,147.32 v135.89,147.32 v138.43,147.32
N$653  (via drill 0.94)
  Bottom 2.032: v128.27,149.86 v130.81,149.86 v133.35,149.86 v135.89,149.86 v138.43,149.86
N$654  (via drill 0.94)
  Bottom 2.032: v128.27,152.4 v130.81,152.4 v133.35,152.4 v135.89,152.4 v138.43,152.4
N$655  (via drill 0.94)
  Bottom 2.032: v128.27,154.94 v130.81,154.94 v133.35,154.94 v135.89,154.94 v138.43,154.94
N$656  (via drill 0.94)
  Bottom 2.032: v128.27,157.48 v130.81,157.48 v133.35,157.48 v135.89,157.48 v138.43,157.48
N$657  (via drill 0.94)
  Bottom 2.032: v128.27,160.02 v130.81,160.02 v133.35,160.02 v135.89,160.02 v138.43,160.02
N$658  (via drill 0.94)
  Bottom 2.032: v128.27,162.56 v130.81,162.56 v133.35,162.56 v135.89,162.56 v138.43,162.56
N$659  (via drill 0.94)
  Bottom 2.032: v128.27,165.1 v130.81,165.1 v133.35,165.1 v135.89,165.1 v138.43,165.1
N$660  (via drill 0.94)
  Bottom 2.032: v128.27,167.64 v130.81,167.64 v133.35,167.64 v135.89,167.64 v138.43,167.64
N$661  (via drill 0.94)
  Bottom 2.032: v128.27,170.18 v130.81,170.18 v133.35,170.18 v135.89,170.18 v138.43,170.18
N$662  (via drill 0.94)
  Bottom 2.032: v128.27,172.72 v130.81,172.72 v133.35,172.72 v135.89,172.72 v138.43,172.72
N$663  (via drill 0.94)
  Bottom 2.032: v128.27,175.26 v130.81,175.26 v133.35,175.26 v135.89,175.26 v138.43,175.26
N$664  (via drill 0.94)
  Bottom 2.032: v128.27,177.8 v130.81,177.8 v133.35,177.8 v135.89,177.8 v138.43,177.8
N$665  (via drill 0.94)
  Bottom 2.032: v128.27,180.34 v130.81,180.34 v133.35,180.34 v135.89,180.34 v138.43,180.34
N$666  (via drill 0.94)
  Bottom 2.032: v128.27,182.88 v130.81,182.88 v133.35,182.88 v135.89,182.88 v138.43,182.88
N$667  (via drill 0.94)
  Bottom 2.032: v128.27,185.42 v130.81,185.42 v133.35,185.42 v135.89,185.42 v138.43,185.42
N$668  (via drill 0.94)
  Bottom 2.032: v128.27,187.96 v130.81,187.96 v133.35,187.96 v135.89,187.96 v138.43,187.96
N$669  (via drill 0.94)
  Bottom 2.032: v128.27,190.5 v130.81,190.5 v133.35,190.5 v135.89,190.5 v138.43,190.5
N$670  (via drill 0.94)
  Bottom 2.032: v128.27,193.04 v130.81,193.04 v133.35,193.04 v135.89,193.04 v138.43,193.04
N$671  (via drill 0.94)
  Bottom 2.032: v128.27,195.58 v130.81,195.58 v133.35,195.58 v135.89,195.58 v138.43,195.58
N$672  (via drill 0.94)
  Bottom 2.032: v128.27,198.12 v130.81,198.12 v133.35,198.12 v135.89,198.12 v138.43,198.12
N$673  (via drill 0.94)
  Bottom 2.032: v128.27,200.66 v130.81,200.66 v133.35,200.66 v135.89,200.66 v138.43,200.66
N$674  (via drill 0.94)
  Bottom 2.032: v128.27,203.2 v130.81,203.2 v133.35,203.2 v135.89,203.2 v138.43,203.2
N$675  (via drill 0.94)
  Bottom 2.032: v128.27,205.74 v130.81,205.74 v133.35,205.74 v135.89,205.74 v138.43,205.74
N$676  (via drill 0.94)
  Bottom 2.032: v128.27,208.28 v130.81,208.28 v133.35,208.28 v135.89,208.28 v138.43,208.28
N$677  (via drill 0.94)
  Bottom 2.032: v128.27,210.82 v130.81,210.82 v133.35,210.82 v135.89,210.82 v138.43,210.82
N$678  (via drill 0.94)
  Bottom 2.032: v128.27,213.36 v130.81,213.36 v133.35,213.36 v135.89,213.36 v138.43,213.36
N$679  (via drill 0.94)
  Bottom 2.032: v128.27,215.9 v130.81,215.9 v133.35,215.9 v135.89,215.9 v138.43,215.9
N$680  (via drill 0.94)
  Bottom 2.032: v128.27,218.44 v130.81,218.44 v133.35,218.44 v135.89,218.44 v138.43,218.44
N$681  (via drill 0.94)
  Bottom 2.032: v128.27,220.98 v130.81,220.98 v133.35,220.98 v135.89,220.98 v138.43,220.98
N$682  (via drill 0.94)
  Bottom 2.032: v128.27,223.52 v130.81,223.52 v133.35,223.52 v135.89,223.52 v138.43,223.52
N$683  (via drill 0.94)
  Bottom 2.032: v128.27,226.06 v130.81,226.06 v133.35,226.06 v135.89,226.06 v138.43,226.06
N$684  (via drill 0.94)
  Bottom 2.032: v128.27,228.6 v130.81,228.6 v133.35,228.6 v135.89,228.6 v138.43,228.6
N$685  (via drill 0.94)
  Bottom 2.032: v128.27,231.14 v130.81,231.14 v133.35,231.14 v135.89,231.14 v138.43,231.14
N$686  (via drill 0.94)
  Bottom 2.032: v128.27,233.68 v130.81,233.68 v133.35,233.68 v135.89,233.68 v138.43,233.68
N$687  (via drill 0.94)
  Bottom 2.032: v128.27,236.22 v130.81,236.22 v133.35,236.22 v135.89,236.22 v138.43,236.22
N$688  (via drill 0.94)
  Bottom 2.032: v128.27,238.76 v130.81,238.76 v133.35,238.76 v135.89,238.76 v138.43,238.76
N$689  (via drill 0.94)
  Bottom 2.032: v128.27,241.3 v130.81,241.3 v133.35,241.3 v135.89,241.3 v138.43,241.3
N$690  (via drill 0.94)
  Bottom 2.032: v128.27,243.84 v130.81,243.84 v133.35,243.84 v135.89,243.84 v138.43,243.84
N$691  (via drill 0.94)
  Bottom 2.032: v128.27,246.38 v130.81,246.38 v133.35,246.38 v135.89,246.38 v138.43,246.38
N$692  (via drill 0.94)
  Bottom 2.032: v128.27,248.92 v130.81,248.92 v133.35,248.92 v135.89,248.92 v138.43,248.92
N$693  (via drill 0.94)
  Bottom 2.032: v128.27,251.46 v130.81,251.46 v133.35,251.46 v135.89,251.46 v138.43,251.46
N$694  (via drill 0.94)
  Bottom 2.032: v128.27,254 v130.81,254 v133.35,254 v135.89,254 v138.43,254
N$695  (via drill 0.94)
  Bottom 2.032: v128.27,256.54 v130.81,256.54 v133.35,256.54 v135.89,256.54 v138.43,256.54
N$696  (via drill 0.94)
  Bottom 2.032: v128.27,259.08 v130.81,259.08 v133.35,259.08 v135.89,259.08 v138.43,259.08
N$697  (via drill 0.94)
  Bottom 2.032: v128.27,261.62 v130.81,261.62 v133.35,261.62 v135.89,261.62 v138.43,261.62
N$698  (via drill 0.94)
  Bottom 2.032: v128.27,264.16 v130.81,264.16 v133.35,264.16 v135.89,264.16 v138.43,264.16
N$699  (via drill 0.94)
  Bottom 2.032: v128.27,266.7 v130.81,266.7 v133.35,266.7 v135.89,266.7 v138.43,266.7
N$700  (via drill 0.94)
  Bottom 2.032: v128.27,269.24 v130.81,269.24 v133.35,269.24 v135.89,269.24 v138.43,269.24
N$701  (via drill 0.94)
  Bottom 2.032: v128.27,271.78 v130.81,271.78 v133.35,271.78 v135.89,271.78 v138.43,271.78
N$702  (via drill 0.94)
  Bottom 2.032: v128.27,274.32 v130.81,274.32 v133.35,274.32 v135.89,274.32 v138.43,274.32
N$703  (via drill 0.94)
  Bottom 2.032: v128.27,276.86 v130.81,276.86 v133.35,276.86 v135.89,276.86 v138.43,276.86
N$704  (via drill 0.94)
  Bottom 2.032: v140.97,12.7 v143.51,12.7 v146.05,12.7 v148.59,12.7 v151.13,12.7
N$705  (via drill 0.94)
  Bottom 2.032: v140.97,15.24 v143.51,15.24 v146.05,15.24 v148.59,15.24 v151.13,15.24
N$706  (via drill 0.94)
  Bottom 2.032: v140.97,17.78 v143.51,17.78 v146.05,17.78 v148.59,17.78 v151.13,17.78
N$707  (via drill 0.94)
  Bottom 2.032: v140.97,20.32 v143.51,20.32 v146.05,20.32 v148.59,20.32 v151.13,20.32
N$708  (via drill 0.94)
  Bottom 2.032: v140.97,22.86 v143.51,22.86 v146.05,22.86 v148.59,22.86 v151.13,22.86
N$709  (via drill 0.94)
  Bottom 2.032: v140.97,25.4 v143.51,25.4 v146.05,25.4 v148.59,25.4 v151.13,25.4
N$710  (via drill 0.94)
  Bottom 2.032: v140.97,27.94 v143.51,27.94 v146.05,27.94 v148.59,27.94 v151.13,27.94
N$711  (via drill 0.94)
  Bottom 2.032: v140.97,30.48 v143.51,30.48 v146.05,30.48 v148.59,30.48 v151.13,30.48
N$712  (via drill 0.94)
  Bottom 2.032: v140.97,33.02 v143.51,33.02 v146.05,33.02 v148.59,33.02 v151.13,33.02
N$713  (via drill 0.94)
  Bottom 2.032: v140.97,35.56 v143.51,35.56 v146.05,35.56 v148.59,35.56 v151.13,35.56
N$714  (via drill 0.94)
  Bottom 2.032: v140.97,38.1 v143.51,38.1 v146.05,38.1 v148.59,38.1 v151.13,38.1
N$715  (via drill 0.94)
  Bottom 2.032: v140.97,40.64 v143.51,40.64 v146.05,40.64 v148.59,40.64 v151.13,40.64
N$716  (via drill 0.94)
  Bottom 2.032: v140.97,43.18 v143.51,43.18 v146.05,43.18 v148.59,43.18 v151.13,43.18
N$717  (via drill 0.94)
  Bottom 2.032: v140.97,45.72 v143.51,45.72 v146.05,45.72 v148.59,45.72 v151.13,45.72
N$718  (via drill 0.94)
  Bottom 2.032: v140.97,48.26 v143.51,48.26 v146.05,48.26 v148.59,48.26 v151.13,48.26
N$719  (via drill 0.94)
  Bottom 2.032: v140.97,50.8 v143.51,50.8 v146.05,50.8 v148.59,50.8 v151.13,50.8
N$720  (via drill 0.94)
  Bottom 2.032: v140.97,53.34 v143.51,53.34 v146.05,53.34 v148.59,53.34 v151.13,53.34
N$721  (via drill 0.94)
  Bottom 2.032: v140.97,55.88 v143.51,55.88 v146.05,55.88 v148.59,55.88 v151.13,55.88
N$722  (via drill 0.94)
  Bottom 2.032: v140.97,58.42 v143.51,58.42 v146.05,58.42 v148.59,58.42 v151.13,58.42
N$723  (via drill 0.94)
  Bottom 2.032: v140.97,60.96 v143.51,60.96 v146.05,60.96 v148.59,60.96 v151.13,60.96
N$724  (via drill 0.94)
  Bottom 2.032: v140.97,63.5 v143.51,63.5 v146.05,63.5 v148.59,63.5 v151.13,63.5
N$725  (via drill 0.94)
  Bottom 2.032: v140.97,66.04 v143.51,66.04 v146.05,66.04 v148.59,66.04 v151.13,66.04
N$726  (via drill 0.94)
  Bottom 2.032: v140.97,68.58 v143.51,68.58 v146.05,68.58 v148.59,68.58 v151.13,68.58
N$727  (via drill 0.94)
  Bottom 2.032: v140.97,71.12 v143.51,71.12 v146.05,71.12 v148.59,71.12 v151.13,71.12
N$728  (via drill 0.94)
  Bottom 2.032: v140.97,73.66 v143.51,73.66 v146.05,73.66 v148.59,73.66 v151.13,73.66
N$729  (via drill 0.94)
  Bottom 2.032: v140.97,76.2 v143.51,76.2 v146.05,76.2 v148.59,76.2 v151.13,76.2
N$730  (via drill 0.94)
  Bottom 2.032: v140.97,78.74 v143.51,78.74 v146.05,78.74 v148.59,78.74 v151.13,78.74
N$731  (via drill 0.94)
  Bottom 2.032: v140.97,81.28 v143.51,81.28 v146.05,81.28 v148.59,81.28 v151.13,81.28
N$732  (via drill 0.94)
  Bottom 2.032: v140.97,83.82 v143.51,83.82 v146.05,83.82 v148.59,83.82 v151.13,83.82
N$733  (via drill 0.94)
  Bottom 2.032: v140.97,86.36 v143.51,86.36 v146.05,86.36 v148.59,86.36 v151.13,86.36
N$734  (via drill 0.94)
  Bottom 2.032: v140.97,88.9 v143.51,88.9 v146.05,88.9 v148.59,88.9 v151.13,88.9
N$735  (via drill 0.94)
  Bottom 2.032: v140.97,91.44 v143.51,91.44 v146.05,91.44 v148.59,91.44 v151.13,91.44
N$736  (via drill 0.94)
  Bottom 2.032: v140.97,93.98 v143.51,93.98 v146.05,93.98 v148.59,93.98 v151.13,93.98
N$737  (via drill 0.94)
  Bottom 2.032: v140.97,96.52 v143.51,96.52 v146.05,96.52 v148.59,96.52 v151.13,96.52
N$738  (via drill 0.94)
  Bottom 2.032: v140.97,99.06 v143.51,99.06 v146.05,99.06 v148.59,99.06 v151.13,99.06
N$739  (via drill 0.94)
  Bottom 2.032: v140.97,101.6 v143.51,101.6 v146.05,101.6 v148.59,101.6 v151.13,101.6
N$740  (via drill 0.94)
  Bottom 2.032: v140.97,104.14 v143.51,104.14 v146.05,104.14 v148.59,104.14 v151.13,104.14
N$741  (via drill 0.94)
  Bottom 2.032: v140.97,106.68 v143.51,106.68 v146.05,106.68 v148.59,106.68 v151.13,106.68
N$742  (via drill 0.94)
  Bottom 2.032: v140.97,109.22 v143.51,109.22 v146.05,109.22 v148.59,109.22 v151.13,109.22
N$743  (via drill 0.94)
  Bottom 2.032: v140.97,111.76 v143.51,111.76 v146.05,111.76 v148.59,111.76 v151.13,111.76
N$744  (via drill 0.94)
  Bottom 2.032: v140.97,114.3 v143.51,114.3 v146.05,114.3 v148.59,114.3 v151.13,114.3
N$745  (via drill 0.94)
  Bottom 2.032: v140.97,116.84 v143.51,116.84 v146.05,116.84 v148.59,116.84 v151.13,116.84
N$746  (via drill 0.94)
